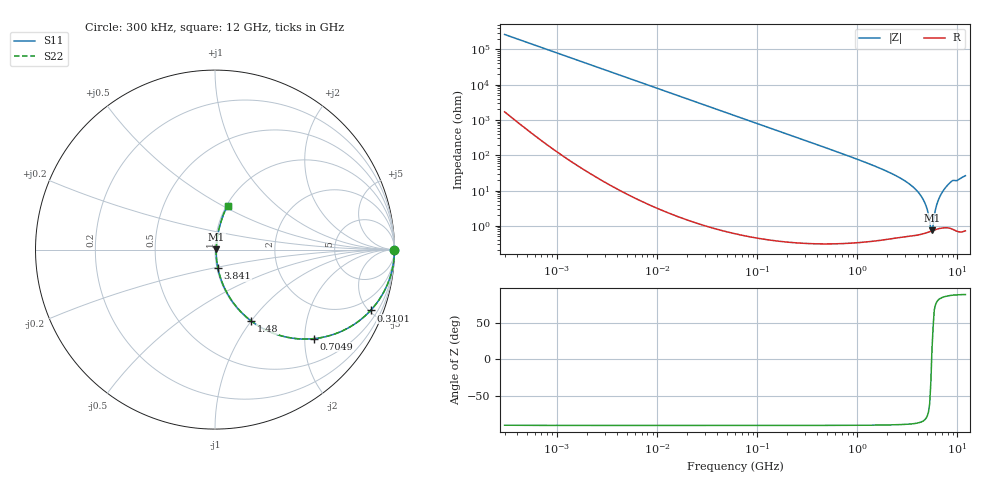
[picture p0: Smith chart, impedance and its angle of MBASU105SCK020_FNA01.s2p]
! MBASU105SCK020_FNA01  S-PARAMETER MODEL  ( Standard Model )
! Model Generated by TAIYO YUDEN Corporation (http://www.ty-top.com)
! Version 1.0
! TAIYO YUDEN Control No. 230609
! Copyright(c) 2023 TAIYO YUDEN CO.,LTD. All Rights Reserved.
! Product Description (link to TY-COMPAS)
! https://ds.yuden.co.jp/TYCOMPAS/or/detail?pn=MBASU105SCK020BFNA01&u=M
! Products Name : Multilayer Ceramic Capacitors
! Characteristics :
!  Capacitance : 2 [pF] , Rated Voltage : 50 [V] , TCC : CK / C0K
!  Case Size : 1.0 x 0.5 / 0.039 x 0.02 [mm/inch] , Thickness : 0.5 / 0.02 [mm/inch]
!  (Conditions: Temperature = 25 [degC] , DC Bias Voltage = 0 [V])
! External Node Assignments :
!  1  o---| |---o  2
! GND o---------o GND
! Frequency Range : 0.3MHz  -  12000MHz  [ 401 STEP ]
# MHZ S RI R 50
! Freq[MHz].  S11 Real  S11 Imag  S21 Real  S21 Imag  S12 Real  S12 Imag  S22 Real  S22 Imag
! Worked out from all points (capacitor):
!   401 points, 300 kHz to 12 GHz, reference 50 ohm
!   read as one part in series: C = 2 pF near 316.3 kHz
!   lowest |Z| = 740 mohm at 5.566 GHz (marker M1)
!   series resonance near 5.524 GHz, so ESL is about 420 pH
!   S11 on the Smith chart (normalised r, x): 300 kHz: open; 310.1 MHz: 1.01, -5.12; 704.9 MHz: 1.01, -2.22; 1.48 GHz: 1.01, -1.00; 3.841 GHz: 1.01, -0.21; 12 GHz: 1.01, +0.53
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0.3  1 -0.000377  2.56e-06 0.000377  2.56e-06 0.000377  1 -0.000377
1.769972  1 -0.00222  7.05e-06 0.00222  7.05e-06 0.00222  1 -0.00222
10.44266  0.9998 -0.0131  0.000177 0.0131  0.000177 0.0131  0.9998 -0.0131
60  0.9943 -0.075  0.00569 0.075  0.00569 0.075  0.9943 -0.075
164.1901  0.959 -0.198  0.041 0.198  0.041 0.198  0.959 -0.198
310.0777  0.8671 -0.3388  0.1329 0.3388  0.1329 0.3388  0.8671 -0.3388
353.9943  0.8333 -0.372  0.1667 0.372  0.1667 0.372  0.8333 -0.372
704.9044  0.552 -0.4959  0.448 0.4959  0.448 0.4959  0.552 -0.4959
1480.043  0.201 -0.397  0.799 0.397  0.799 0.397  0.201 -0.397
2088.533  0.0992 -0.2925  0.9008 0.2925  0.9008 0.2925  0.0992 -0.2925
2947.191  0.04 -0.1839  0.96 0.1839  0.96 0.1839  0.04 -0.1839
3841.137  0.0163 -0.1039  0.9837 0.1039  0.9837 0.1039  0.0163 -0.1039
4623.766  0.0085 -0.0498  0.9915 0.0498  0.9915 0.0498  0.0085 -0.0498
4875.354  0.00748 -0.0346  0.9925 0.0346  0.9925 0.0346  0.00748 -0.0346
5278.635  0.0069 -0.0118  0.9931 0.0118  0.9931 0.0118  0.0069 -0.0118
5420.343  0.00696 -0.00423  0.993 0.00423  0.993 0.00423  0.00696 -0.00423
5565.855  0.00714 0.00174  0.9929 -0.00174  0.9929 -0.00174  0.00714 0.00174
5715.274  0.00738 0.00717  0.9926 -0.00717  0.9926 -0.00717  0.00738 0.00717
6354.153  0.0103 0.0468  0.9897 -0.0468  0.9897 -0.0468  0.0103 0.0468
7254.098  0.0186 0.0986  0.9814 -0.0986  0.9814 -0.0986  0.0186 0.0986
8732.115  0.0397 0.1741  0.9603 -0.1741  0.9603 -0.1741  0.0397 0.1741
12000  0.0708 0.2432  0.9292 -0.2432  0.9292 -0.2432  0.0708 0.2432
